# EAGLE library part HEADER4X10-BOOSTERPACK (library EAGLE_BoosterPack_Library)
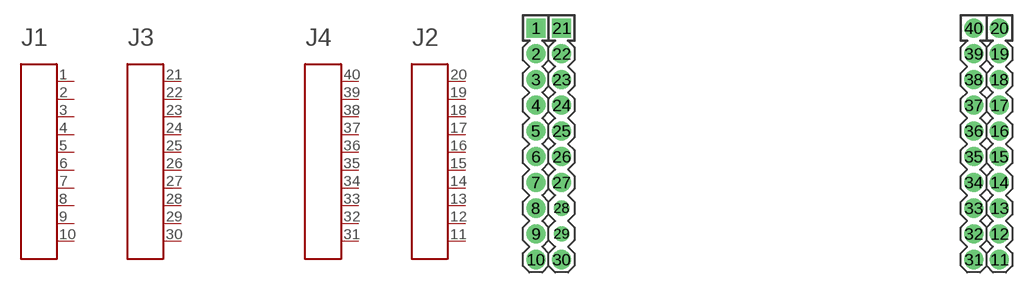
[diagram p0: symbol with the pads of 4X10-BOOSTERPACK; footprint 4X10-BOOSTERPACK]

Designator prefix A

## HEADER4X10-BOOSTERPACK  [4X10-BOOSTERPACK]
1  P$1
2  P$2
3  P$3
4  P$4
5  P$5
6  P$6
7  P$7
8  P$8
9  P$9
10  P$10
11  P$11
12  P$12
13  P$13
14  P$14
15  P$15
16  P$16
17  P$17
18  P$18
19  P$19
20  P$20
21  P$21
22  P$22
23  P$23
24  P$24
25  P$25
26  P$26
27  P$27
28  P$28
29  P$29
30  P$30
31  P$31
32  P$32
33  P$33
34  P$34
35  P$35
36  P$36
37  P$37
38  P$38
39  P$39
40  P$40

## Footprint 4X10-BOOSTERPACK (pad centres in mm)
drill 1.016 pad 1.88 square: 1 0,10.16; 21 2.54,10.16
drill 1.016 pad 1.88: 2 0,7.62; 3 0,5.08; 4 0,2.54; 5 0,0; 6 0,-2.54; 7 0,-5.08; 8 0,-7.62; 9 0,-10.16; 10 0,-12.7; 11 45.72,-12.7; 12 45.72,-10.16; 13 45.72,-7.62; 14 45.72,-5.08; 15 45.72,-2.54; 16 45.72,0; 17 45.72,2.54; 18 45.72,5.08; 19 45.72,7.62; 20 45.72,10.16; 22 2.54,7.62; 23 2.54,5.08; 24 2.54,2.54; 25 2.54,0; 26 2.54,-2.54; 27 2.54,-5.08; 30 2.54,-12.7; 31 43.18,-12.7; 32 43.18,-10.16; 33 43.18,-7.62; 34 43.18,-5.08; 35 43.18,-2.54; 36 43.18,0; 37 43.18,2.54; 38 43.18,5.08; 39 43.18,7.62; 40 43.18,10.16
drill 1.016 pad 1.422: 28 2.54,-7.62; 29 2.54,-10.16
